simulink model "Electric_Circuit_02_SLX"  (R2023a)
settings: Solver=ode23s  StartTime=0.0  StopTime=10.0  MaxStep=0.001  RelTol=1e-3
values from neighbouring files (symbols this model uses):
  C_5 = 0.001*F    (= 0.001)    [Electric_Circuit_02_EQN.m]    (also in Electric_Circuit_02_SLX_m.m; Electric_Circuit_04_EQN.m; Electric_Circuit_04_SLX_m.m; Electric_Circuit_05_EQN.m)
  C_7 = 0.001*F    (= 0.001)    [Electric_Circuit_02_EQN.m]    (also in Electric_Circuit_02_SLX_m.m; Electric_Circuit_04_EQN.m; Electric_Circuit_04_SLX_m.m; Electric_Circuit_05_EQN.m)
  I_2_0 = 0*A    (= 0)    [Electric_Circuit_02_SLX_m.m]    (also in Electric_Circuit_03_SLX_m.m; Electric_Circuit_06_SLX_m.m; Electric_Circuit_08_SLX_m.m; Electric_Circuit_09_SLX_m.m)
  I_4_0 = 0*A    (= 0)    [Electric_Circuit_02_SLX_m.m]    (also in Electric_Circuit_03_SLX_m.m; Electric_Circuit_04_SLX_m.m; Electric_Circuit_05_SLX_m.m; Electric_Circuit_07_SLX_m.m)
  I_8_0 = 0*A    (= 0)    [Electric_Circuit_02_SLX_m.m]    (also in Electric_Circuit_05_SLX_m.m; Electric_Circuit_06_SLX_m.m; Electric_Circuit_07_SLX_m.m; Electric_Circuit_08_SLX_m.m)
  L_2 = 0.002*H    (= 0.002)    [Electric_Circuit_02_EQN.m]    (also in Electric_Circuit_02_SLX_m.m; Electric_Circuit_03_EQN.m; Electric_Circuit_03_SLX_m.m; Electric_Circuit_06_EQN.m)
  L_4 = 0.002*H    (= 0.002)    [Electric_Circuit_02_EQN.m]    (also in Electric_Circuit_02_SLX_m.m; Electric_Circuit_03_EQN.m; Electric_Circuit_03_SLX_m.m; Electric_Circuit_04_EQN.m)
  R_3 = 100*Ohm    (= 100)    [Electric_Circuit_02_EQN.m]    (also in Electric_Circuit_02_SLX_m.m; Electric_Circuit_01_EQN.m; Electric_Circuit_01_SLX_m.m; Electric_Circuit_04_EQN.m)
  R_6 = 100*Ohm    (= 100)    [Electric_Circuit_02_EQN.m]    (also in Electric_Circuit_02_SLX_m.m; BIG_EC_Simscape_EQN.m; BIG_EC_Simscape_SLX_m.m; Electric_Circuit_04_EQN.m)
  Ts = Tfin/Nr_Ts_Points    (= 0.000480145)    [Electric_Circuit_02_SLX_m.m]    (also in BIG_EC_Simscape_SLX_m.m = 0.0003; Car_Dumper_SLX_m.m = 0.0022779; Electric_Circuit_01_SLX_m.m = 0.005; Electric_Circuit_03_SLX_m.m = 0.0006)
  V_1_0 = 10*V    (= 10)    [Electric_Circuit_02_SLX_m.m]    (also in BIG_EC_Simscape_SLX_m.m; Electric_Circuit_03_SLX_m.m; Electric_Circuit_04_SLX_m.m; Electric_Circuit_05_SLX_m.m)
  V_5_0 = 0*V    (= 0)    [Electric_Circuit_02_SLX_m.m]    (also in Electric_Circuit_04_SLX_m.m; Electric_Circuit_05_SLX_m.m; Electric_Circuit_08_SLX_m.m)
  V_7_0 = 0*V    (= 0)    [Electric_Circuit_02_SLX_m.m]    (also in Electric_Circuit_04_SLX_m.m; Electric_Circuit_05_SLX_m.m; Electric_Circuit_07_SLX_m.m; Electric_Circuit_10_SLX_m.m)

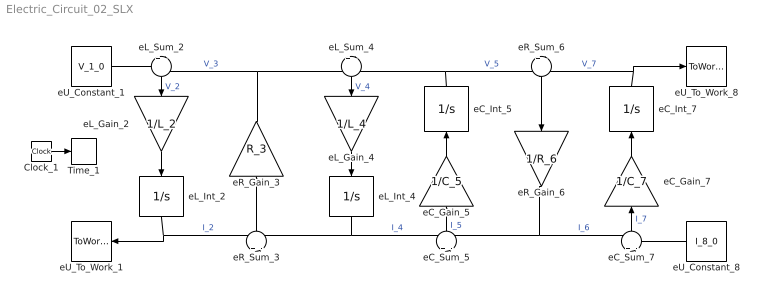
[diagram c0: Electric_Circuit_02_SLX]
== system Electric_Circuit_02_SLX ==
  Clock_1 : Clock
  Time_1 : ToWorkspace  VariableName=t  SaveFormat=Timeseries  SampleTime=Ts
  eC_Gain_5 : Gain  Gain=1/C_5  Multiplication=Matrix(K*u)
  eC_Gain_7 : Gain  Gain=1/C_7  Multiplication=Matrix(K*u)
  eC_Int_5 : Integrator  InitialCondition=V_5_0
  eC_Int_7 : Integrator  InitialCondition=V_7_0
  eC_Sum_5 : Sum  Inputs=+|-
  eC_Sum_7 : Sum  Inputs=+|-
  eL_Gain_2 : Gain  Gain=1/L_2  Multiplication=Matrix(K*u)
  eL_Gain_4 : Gain  Gain=1/L_4  Multiplication=Matrix(K*u)
  eL_Int_2 : Integrator  InitialCondition=I_2_0
  eL_Int_4 : Integrator  InitialCondition=I_4_0
  eL_Sum_2 : Sum  Inputs=+|-
  eL_Sum_4 : Sum  Inputs=+|-
  eR_Gain_3 : Gain  Gain=R_3  Multiplication=Matrix(K*u)
  eR_Gain_6 : Gain  Gain=1/R_6  Multiplication=Matrix(K*u)
  eR_Sum_3 : Sum  Inputs=+|-
  eR_Sum_6 : Sum  Inputs=+|-
  eU_Constant_1 : Constant  Value=V_1_0
  eU_Constant_8 : Constant  Value=I_8_0
  eU_To_Work_1 : ToWorkspace  VariableName=I_1_0  SaveFormat=Timeseries  SampleTime=Ts
  eU_To_Work_8 : ToWorkspace  VariableName=V_8_0  SaveFormat=Timeseries  SampleTime=Ts
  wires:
  eU_Constant_1/1 -> eL_Sum_2/1
  eR_Gain_3/1 -> eL_Sum_2/2, eL_Sum_4/1  "V_3"
  eL_Int_2/1 -> eU_To_Work_1/1, eR_Sum_3/1  "I_2"
  eL_Sum_2/1 -> eL_Gain_2/1  "V_2"
  eL_Gain_2/1 -> eL_Int_2/1
  eL_Int_4/1 -> eR_Sum_3/2, eC_Sum_5/1  "I_4"
  eR_Sum_3/1 -> eR_Gain_3/1
  eC_Int_5/1 -> eL_Sum_4/2, eR_Sum_6/1  "V_5"
  eL_Sum_4/1 -> eL_Gain_4/1  "V_4"
  eL_Gain_4/1 -> eL_Int_4/1
  eR_Gain_6/1 -> eC_Sum_5/2, eC_Sum_7/1  "I_6"
  eC_Sum_5/1 -> eC_Gain_5/1  "I_5"
  eC_Gain_5/1 -> eC_Int_5/1
  eC_Int_7/1 -> eR_Sum_6/2, eU_To_Work_8/1  "V_7"
  eR_Sum_6/1 -> eR_Gain_6/1
  eU_Constant_8/1 -> eC_Sum_7/2
  eC_Sum_7/1 -> eC_Gain_7/1  "I_7"
  eC_Gain_7/1 -> eC_Int_7/1
  Clock_1/1 -> Time_1/1
